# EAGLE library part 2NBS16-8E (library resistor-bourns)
BOURNS RESISTOR NETWORK
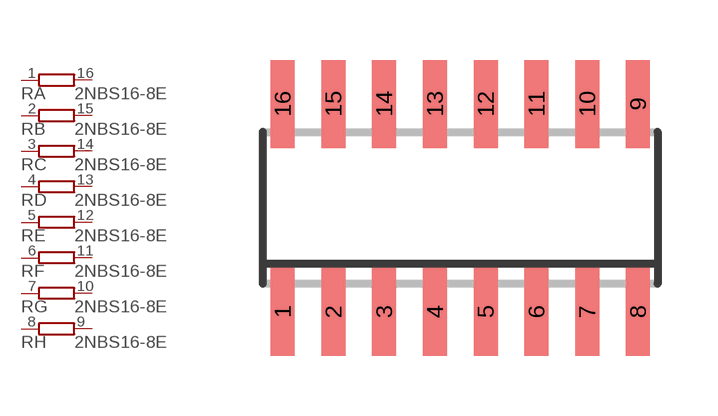
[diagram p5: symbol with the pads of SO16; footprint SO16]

Designator prefix R; gates A=R1NV B=R1NV C=R1NV D=R1NV E=R1NV F=R1NV G=R1NV H=R1NV

## 2NBS16-8E (OC_FARNELL: unknown; OC_NEWARK: unknown)  [SO16]
1  A:1  pas
2  B:1  pas
3  C:1  pas
4  D:1  pas
5  E:1  pas
6  F:1  pas
7  G:1  pas
8  H:1  pas
9  H:2  pas
10  G:2  pas
11  F:2  pas
12  E:2  pas
13  D:2  pas
14  C:2  pas
15  B:2  pas
16  A:2  pas

## Footprint SO16 (pad centres in mm)
BOURNS RESISTOR NETWORK
smd 0.6 x 2.2: 1 -4.445,-2.6; 2 -3.175,-2.6; 3 -1.905,-2.6; 4 -0.635,-2.6; 5 0.635,-2.6; 6 1.905,-2.6; 7 3.175,-2.6; 8 4.445,-2.6; 9 4.445,2.6; 10 3.175,2.6; 11 1.905,2.6; 12 0.635,2.6; 13 -0.635,2.6; 14 -1.905,2.6; 15 -3.175,2.6; 16 -4.445,2.6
